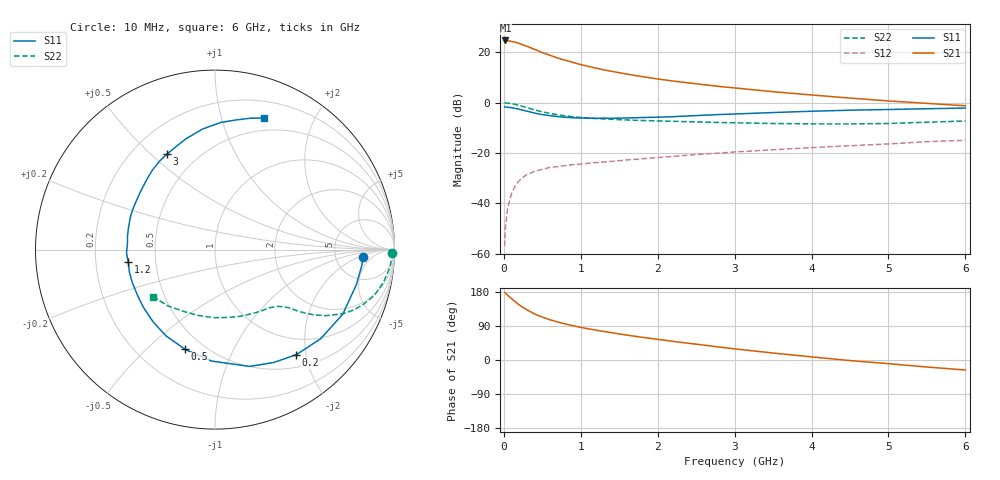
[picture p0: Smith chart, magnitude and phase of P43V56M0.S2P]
! SIEMENS Small Signal Semiconductors
! BFP182
! Si NPN RF Bipolar Junction Transistor in SOT143
! VCE = 3.5 V  IC = 6 mA
! Common Emitter S-Parameters:  March  1996
# GHz  S  MA  R  50
!  f  S11  S21  S12  S22
! GHz  MAG  ANG  MAG  ANG  MAG  ANG  MAG  ANG
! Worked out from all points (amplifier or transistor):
!   36 points, 10 MHz to 6 GHz, reference 50 ohm
!   highest |S21| = 24.8 dB at 20 MHz (marker M1)
!   |S21| within 3 dB of that: start of sweep to 355.4 MHz
!   unconditionally stable (mu >= 1): 1.48 GHz to 5.486 GHz
!   at 250 MHz: K = 0.25, MSG = 26.3 dB, |S12| = -29.7 dB
!   at 1.4 GHz: K = 0.97, MSG = 17.9 dB, |S12| = -23.3 dB
!   at 6 GHz: K = 0.93, MSG = 6.9 dB, |S12| = -14.9 dB
!   lowest NFmin = 1.25 dB at 450 MHz
!   S11 on the Smith chart (normalised r, x): 10 MHz: 10, -2; 200 MHz: 0.70, -1.82; 500 MHz: 0.40, -0.67; 1.2 GHz: 0.35, -0.06; 3 GHz: 0.34, +0.56; 6 GHz: 0.36, +1.38
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0.01  0.8245 -2.7  17.12 178.2  0.0014 83.2  0.9886 -1.0
0.02  0.8237 -5.7  17.3 176.7  0.0033 86.0  0.9854 -2.3
0.05  0.8117 -13.9  17.21 170.7  0.0082 85.7  0.9807 -5.6
0.1  0.7976 -26.9  16.48 161.9  0.0153 74.4  0.9557 -11.0
0.15  0.77 -40.2  15.94 153.3  0.0227 69.2  0.9239 -16.0
0.2  0.7403 -52.3  15.13 145.4  0.0281 64.8  0.8822 -20.2
0.25  0.7085 -62.7  14.06 138.6  0.0329 59.0  0.8404 -23.7
0.3  0.6787 -73.5  13.24 132.5  0.0374 55.6  0.7971 -26.6
0.4  0.6213 -91.8  11.5 121.5  0.0431 49.3  0.7195 -30.8
0.5  0.5803 -106.7  9.913 113.1  0.0474 44.7  0.6578 -33.5
0.6  0.5527 -119.6  8.773 106.2  0.0516 41.7  0.6129 -35.2
0.7  0.53 -130.7  7.727 100.3  0.0535 40.1  0.5762 -36.5
0.8  0.5122 -141.3  6.981 94.9  0.0561 38.4  0.5476 -37.4
1.1  0.4932 -165.1  5.28 82.2  0.0626 37.0  0.4951 -40.0
1.2  0.4881 -171.9  4.858 78.8  0.0644 36.2  0.4848 -40.9
1.7  0.5019 161.2  3.491 62.8  0.0744 36.6  0.4468 -46.3
2.2  0.5276 141.4  2.703 49.1  0.0856 36.0  0.4267 -53.4
3  0.596 116.7  1.968 29.4  0.1046 33.4  0.3987 -68.2
3.5  0.6372 105.0  1.654 18.4  0.1158 31.0  0.3853 -79.1
4.5  0.7095 87.3  1.236 -1.5  0.1395 25.4  0.3785 -104.0
5.5  0.7579 75.0  0.97 -18.5  0.1678 19.6  0.4091 -130.0
6  0.7823 69.5  0.869 -26.4  0.1792 15.2  0.4323 -142.6
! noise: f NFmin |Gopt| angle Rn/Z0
0.45  1.25  0.25  39  0.3
0.9  1.4  0.25  78  0.23
1.8  1.95  0.21  151  0.2
